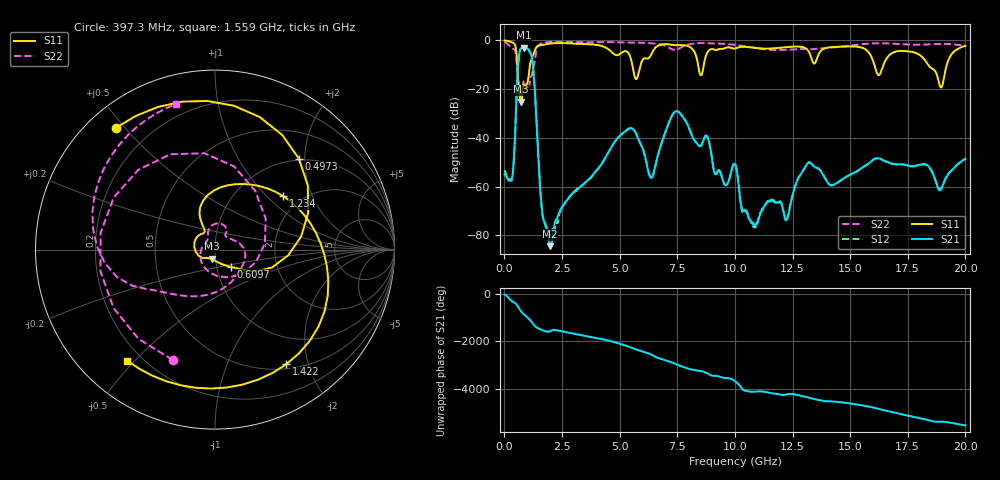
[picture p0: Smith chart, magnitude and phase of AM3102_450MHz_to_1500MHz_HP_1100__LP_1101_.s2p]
!Agilent Technologies,E8364B,MY43040894,A.07.50.67
!Agilent E8364B: A.07.50.67
!Date: Thursday, January 11, 2018 06:35:50
!Correction: S11(Full 2 Port(1,2))
!S21(Full 2 Port(1,2))
!S12(Full 2 Port(1,2))
!S22(Full 2 Port(1,2))
!S2P File: Measurements: S11, S21, S12, S22:
# Hz S  dB  R 50
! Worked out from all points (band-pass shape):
!   1601 points, 10 MHz to 20 GHz, reference 50 ohm
!   highest |S21| = -3.01 dB at 847.1 MHz (marker M1); lowest = -84.5 dB at 1.972 GHz (marker M2)
!   |S21| within 3 dB of the highest: 641.4 MHz to 1.163 GHz (522.1 MHz wide, 57.9 % of centre)
!   lowest |S11| = -25.2 dB at 722.1 MHz (marker M3), VSWR 1.12, Z = 47.9 - j4.91 ohm
!   |S11| at or under -10 dB: 562 MHz to 1.114 GHz (552.3 MHz wide, 65.9 % of centre); 16.05 GHz to 16.45 GHz (401 MHz wide, 2.47 % of centre); 18.38 GHz to 19.2 GHz (820.4 MHz wide, 4.37 % of centre)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
!   |S22| runs from -23.6 to -0.6 dB; largest |S21 - S12| = 0.0064
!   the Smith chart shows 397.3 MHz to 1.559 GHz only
!   S11 on the Smith chart (normalised r, x): 397.3 MHz: 0.08, +0.47; 497.3 MHz: 0.97, +1.88; 609.7 MHz: 1.17, -0.23; 1.234 GHz: 1.62, +1.26; 1.422 GHz: 0.56, -1.66; 1.559 GHz: 0.15, -0.48
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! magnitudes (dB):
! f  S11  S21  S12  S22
! 10 MHz  -0.1  -55.0  -53.3  -0.7
! 397.3 MHz  -1.2  -51.0  -51.0  -3.6
! 497.3 MHz  -3.2  -31.0  -31.0  -5.4
! 609.7 MHz  -17.6  -9.0  -9.0  -17.6
! 722.1 MHz  -25.2  -3.4  -3.4  -23.2
! 847.1 MHz  -18.2  -3.0  -3.0  -16.7
! 1.234 GHz  -6.3  -10.0  -10.0  -12.5
! 1.422 GHz  -2.5  -38.5  -38.5  -2.9
! 1.559 GHz  -2.1  -61.3  -61.7  -1.5
! 1.972 GHz  -1.4  -84.5  -80.1  -0.7
! 3.346 GHz  -1.5  -59.6  -59.7  -0.8
! 5.407 GHz  -5.6  -36.2  -36.2  -1.0
! 6.344 GHz  -6.3  -56.3  -56.2  -1.2
! 6.682 GHz  -2.2  -46.5  -46.6  -1.5
! 7.494 GHz  -2.0  -29.1  -29.1  -3.8
! 9.568 GHz  -3.3  -59.3  -59.1  -1.5
! 10.01 GHz  -3.4  -50.8  -50.7  -1.9
! 10.87 GHz  -3.1  -75.9  -76.7  -3.1
! 13.34 GHz  -8.0  -50.9  -50.8  -3.7
! 16.68 GHz  -6.4  -50.2  -50.3  -1.3
! 18.94 GHz  -19.4  -61.3  -60.8  -1.5
! 20 GHz  -2.3  -48.7  -48.6  -2.3
